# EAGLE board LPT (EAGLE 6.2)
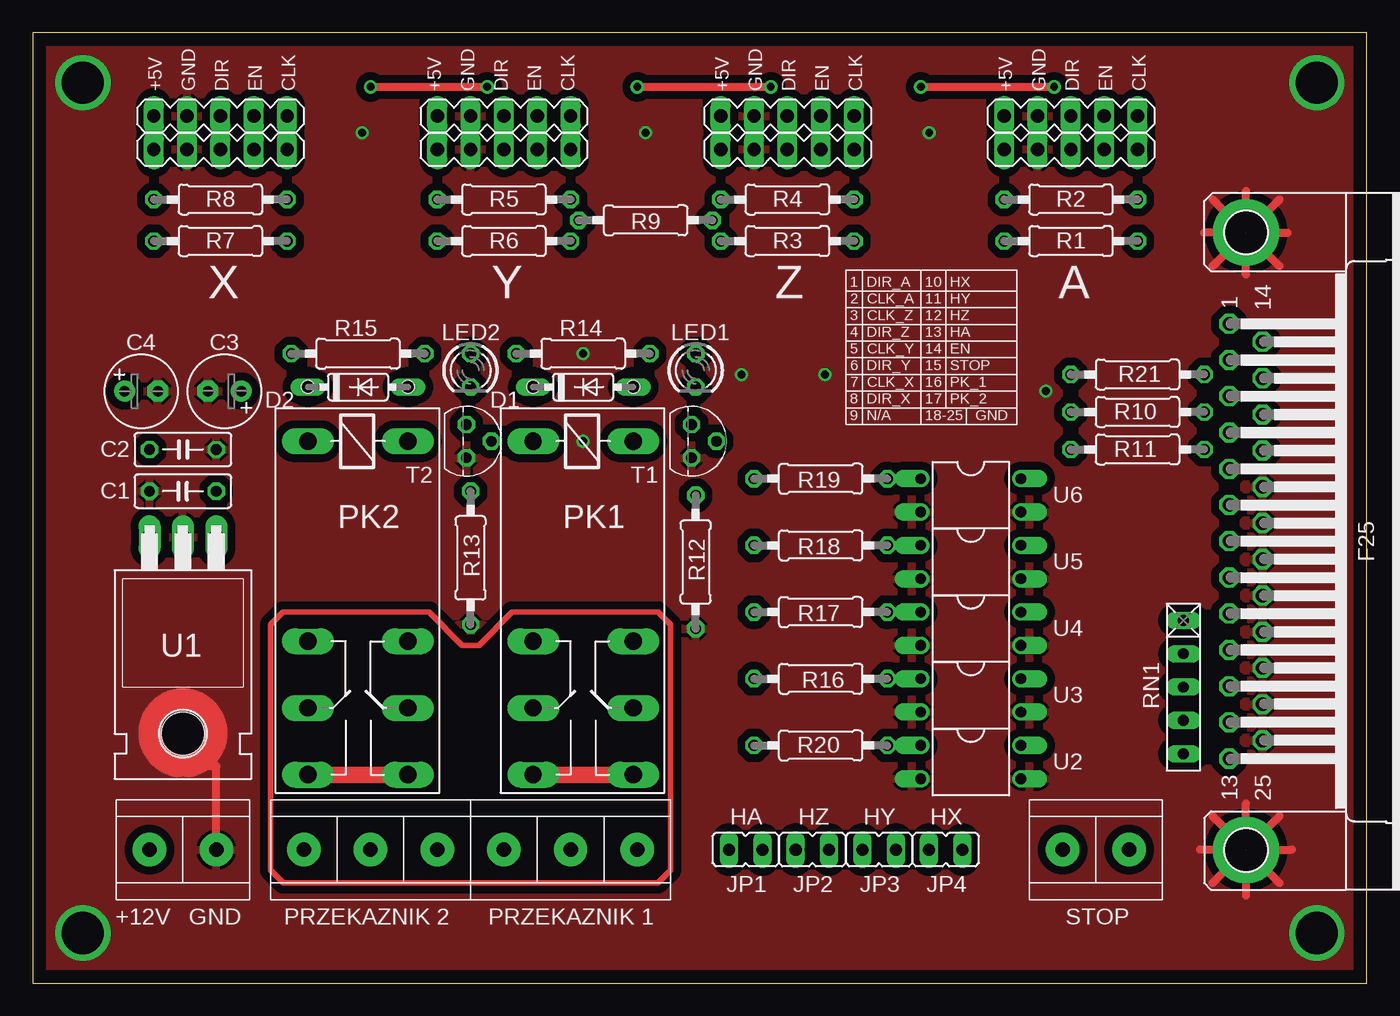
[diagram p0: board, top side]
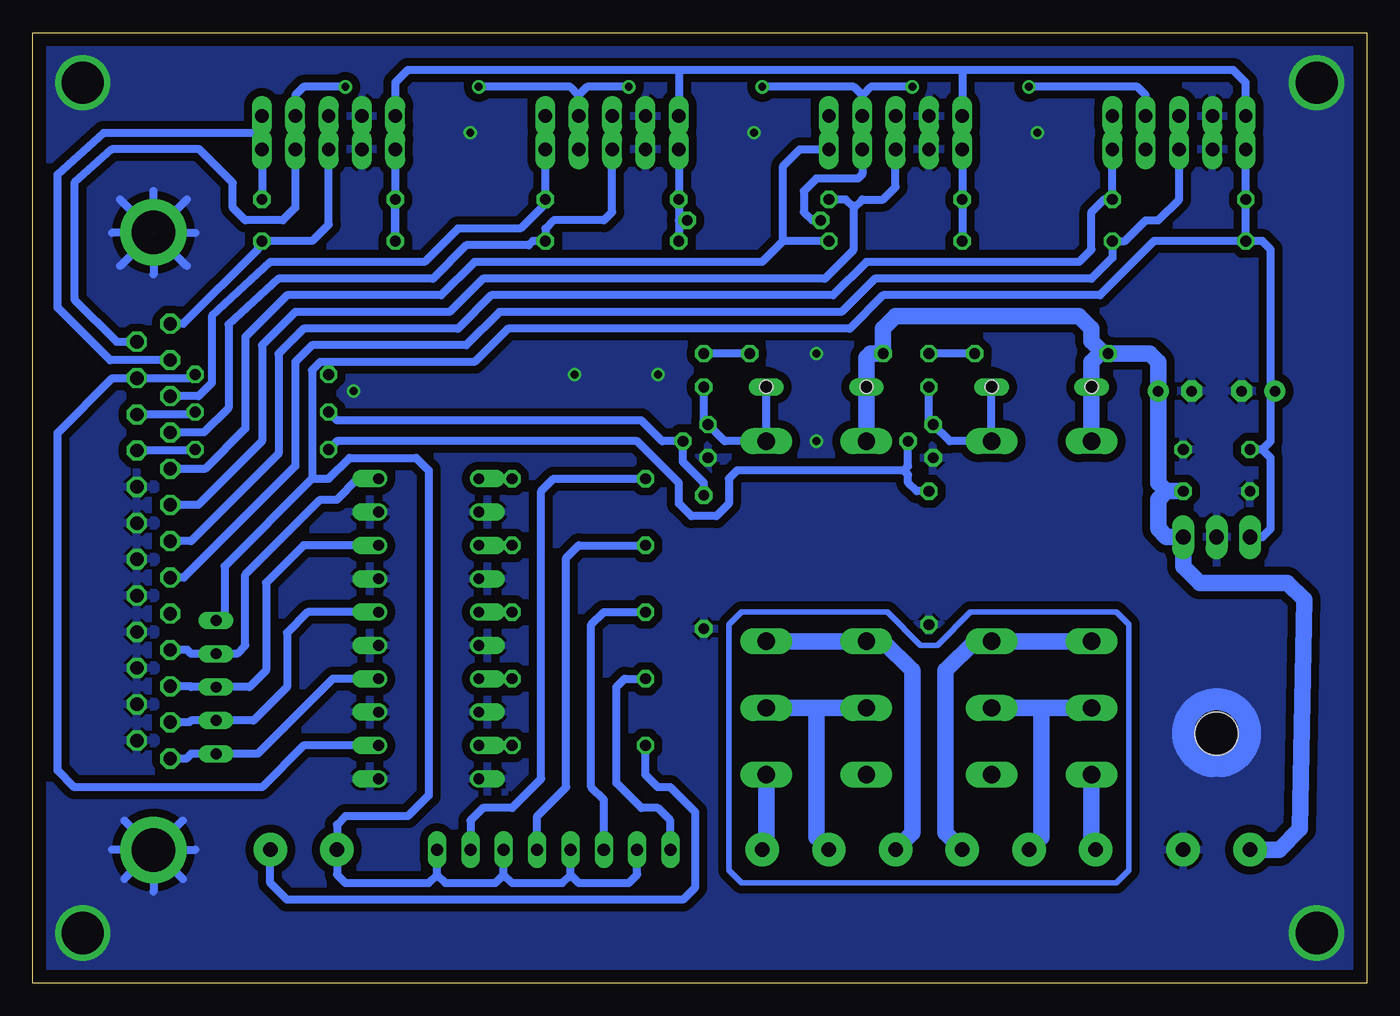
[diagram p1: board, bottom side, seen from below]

Size 101.59 x 72.38 mm. Coordinates in mm from the lower left corner, seen from the top.
Outline: 0,0 101.59,0 101.59,72.38 0,72.38 0,0
Copper layers (1*16): Top 0.035mm / dielectric 1.5mm / Bottom 0.035mm
Design rules: minimum track width 10mil, minimum drill 24mil, track to track 8mil, track to pad 8mil, pad to pad 8mil, via to via 8mil, smd to smd 8mil, copper to edge 40mil, drill to drill 8mil, minimum pad ring 10mil, minimum via ring 8mil, stop-mask expansion 4mil, vias tented up to drill 0mil, thermal gap 10mil
Holes 1 mm at 20.96,45.4 28.57,45.4 38.1,45.4 45.72,45.4

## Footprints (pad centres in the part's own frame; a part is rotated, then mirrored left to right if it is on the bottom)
MA05-1 = drill 1.016 long: 1 -5.08,0; 2 -2.54,0; 3 0,0; 4 2.54,0; 5 5.08,0
C050-025X075 = drill 0.813 octagon: 1 -2.54,0; 2 2.54,0
E2,5-6 = drill 0.813 pad 1.6: + -1.27,0 | drill 0.813 pad 1.6 octagon: - 1.27,0
DO35-7 = drill 0.813 long: A 3.81,0; C -3.81,0
JP1 = drill 0.914 long: 1 0,-1.27; 2 0,1.27
LED3MM = drill 0.813 octagon: A -1.27,0; K 1.27,0
F25HP = drill 1.016 octagon: 1 -16.561,-1.27; 2 -13.792,-1.27; 3 -11.049,-1.27; 4 -8.28,-1.27; 5 -5.512,-1.27; 6 -2.769,-1.27; 7 0,-1.27; 8 2.769,-1.27; 9 5.512,-1.27; 10 8.28,-1.27; 11 11.049,-1.27; 12 13.792,-1.27; 13 16.561,-1.27; 14 -15.189,1.27; 15 -12.421,1.27; 16 -9.652,1.27; 17 -6.909,1.27; 18 -4.14,1.27; 19 -1.372,1.27; 20 1.372,1.27; 21 4.14,1.27; 22 6.909,1.27; 23 9.652,1.27; 24 12.421,1.27; 25 15.189,1.27 | drill 3.302 pad 5.08: G1 -23.52,0; GND 23.52,0
F4052 = drill 1.321 long: 1 -3.81,3.81; 2 -3.81,-3.81; O1 11.43,-3.81; O2 11.43,3.81; P1 16.51,-3.81; P2 16.51,3.81; S1 21.59,-3.81; S2 21.59,3.81
0207/10 = drill 0.813 octagon: 1 -5.08,0; 2 5.08,0
RN-5 = drill 0.813 long: 1 -5.08,0; 2 -2.54,0; 3 0,0; 4 2.54,0; 5 5.08,0
TO92 = drill 0.813 octagon: 1 1.27,0; 2 0,1.905; 3 -1.27,0
TO220H = drill 1.118 long: 1 -2.54,-10.16; 2 0,-10.16; 3 2.54,-10.16 | hole 3.302: 0,4.826
DIL04 = drill 0.813 offset: 1 -1.27,-3.81; 2 1.27,-3.81; 3 1.27,3.81; 4 -1.27,3.81
AREK3 = drill 1.1 pad 2.54: P$1 0,0; P$2 -5.08,0; P$3 5.08,0
ARK2 = drill 1.1 pad 2.54: P$1 -2.54,0; P$2 2.54,0

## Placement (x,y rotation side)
A  [MA05-1]  79.06,63.5 0 top
C1  100nF  [C050-025X075]  11.43,37.46 180 top
C2  100nF  [C050-025X075]  11.43,40.64 0 top
C3  100uF  [E2,5-6]  14.61,45.09 180 top
C4  100uF  [E2,5-6]  8.25,45.09 0 top
D1  1N4148DO35-7  [DO35-7]  41.91,45.4 0 top
D2  1N4148DO35-7  [DO35-7]  24.77,45.4 0 top
JP1  [JP1]  54.29,10.16 270 top
JP2  [JP1]  59.37,10.16 270 top
JP3  [JP1]  64.45,10.16 270 top
JP4  [JP1]  69.53,10.16 270 top
LED1  [LED3MM]  50.48,46.67 270 top
LED2  [LED3MM]  33.34,46.67 270 top
LPT  [F25HP]  92.39,33.66 270 top
PK1  4052  [F4052]  41.91,37.46 270 top
PK2  4052  [F4052]  24.77,37.46 270 top
R1  [0207/10]  79.06,56.52 180 top
R2  [0207/10]  79.06,59.69 180 top
R3  [0207/10]  57.47,56.52 180 top
R4  [0207/10]  57.47,59.69 180 top
R5  [0207/10]  35.88,59.69 180 top
R6  [0207/10]  35.88,56.52 180 top
R7  [0207/10]  14.29,56.52 180 top
R8  [0207/10]  14.29,59.69 180 top
R9  [0207/10]  46.67,58.1 0 top
R10  4,7k  [0207/10]  84.14,43.5 180 top
R11  4,7k  [0207/10]  84.14,40.64 180 top
R12  10k  [0207/10]  50.48,32.07 90 top
R13  10k  [0207/10]  33.34,32.38 90 top
R14  1k  [0207/10]  41.91,47.94 180 top
R15  1k  [0207/10]  24.77,47.94 180 top
R16  330  [0207/10]  60.01,23.18 0 top
R17  330  [0207/10]  60.01,28.26 0 top
R18  330  [0207/10]  60.01,33.34 0 top
R19  330  [0207/10]  60.01,38.42 0 top
R20  330  [0207/10]  60.01,18.1 0 top
R21  4,7k  [0207/10]  84.14,46.35 180 top
RN1  4x4,7k  [RN-5]  87.63,22.54 270 top
S5  [MA05-1]  14.29,66.04 0 top
S6  [MA05-1]  35.88,66.04 0 top
S7  [MA05-1]  57.47,66.04 0 top
S8  [MA05-1]  79.06,66.04 0 top
T1  BC547  [TO92]  50.17,41.27 270 top
T2  BC547  [TO92]  33.02,41.27 270 top
U1  7805T  [TO220H]  11.43,23.81 180 top
U2  PC817  [DIL04]  71.44,16.83 270 top
U3  PC817  [DIL04]  71.44,21.91 270 top
U4  PC817  [DIL04]  71.44,26.99 270 top
U5  PC817  [DIL04]  71.44,32.07 270 top
U6  PC817  [DIL04]  71.44,37.15 270 top
U$2  AREK3  [AREK3]  40.96,10.16 180 top
U$3  AREK3  [AREK3]  25.72,10.16 0 top
U$5  ARK2  [ARK2]  80.96,10.16 180 top
U$7  ARK2  [ARK2]  11.43,10.16 0 top
X  [MA05-1]  14.29,63.5 0 top
Y  [MA05-1]  35.88,63.5 0 top
Z  [MA05-1]  57.47,63.5 0 top

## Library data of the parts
A S5-S8 X Y Z = con-lstb
C1-C4 R1-R21 = rcl
D1 D2 = diode
JP1-JP4 = jumper
LED1 LED2 = led
LPT = con-subd
PK1 PK2 = relay
RN1 = resistor-net
T1 T2 = transistor-npn
U1 = linear
U2-U6 = optocoupler
U$2 U$3 = arek3
U$5 U$7 = !ark2m

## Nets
GND: A.2 C1.2 C2.2 C3.- C4.- LPT.18 LPT.19 LPT.20 LPT.21 LPT.22 LPT.23 LPT.24 LPT.25 R12.1 R13.1 S5.2 S6.2 S7.2 S8.2 T1.1 T2.1 U1.2 U2.2 U2.3 U3.2 U3.3 U4.2 U4.3 U5.2 U5.3 U6.2 U6.3 U$7.P$2 X.2 Y.2 Z.2
N$1: D1.A LED1.K PK1.1 T1.3
N$2: D2.A LED2.K PK2.1 T2.3
N$3: LPT.5 R6.1 S6.5 Y.5
N$4: LPT.6 R5.1 S6.3 Y.3
N$5: LPT.8 R7.1 S5.3 X.3
N$6: LPT.4 R3.1 S7.3 Z.3
N$7: A.5 LPT.2 R2.1 S8.5
N$9: PK1.S1 PK1.S2 U$2.P$2
N$10: A.4 LPT.14 R9.1 S5.4 S6.4 S7.4 S8.4 X.4 Y.4 Z.4
N$11: A.3 LPT.1 R1.1 S8.3
N$12: LPT.7 R8.1 S5.5 X.5
N$13: LPT.3 R4.1 S7.5 Z.5
N$14: PK1.O1 PK1.O2 U$2.P$3
N$15: A.1 C2.1 C4.+ JP1.2 JP2.2 JP3.2 JP4.2 R1.2 R2.2 R3.2 R4.2 R5.2 R6.2 R7.2 R8.2 R9.2 R21.2 RN1.1 S5.1 S6.1 S7.1 S8.1 U1.3 U$5.P$2 X.1 Y.1 Z.1
N$16: R10.2 R12.2 T1.2
N$17: R11.2 R13.2 T2.2
N$18: LED1.A R14.1
N$19: LED2.A R15.1
N$20: LPT.16 R10.1
N$21: LPT.17 R11.1
N$24: LPT.15 R21.1 U2.4
N$25: LPT.10 RN1.2 U6.4
N$26: PK2.S1 PK2.S2 U$3.P$2
N$27: PK2.O1 PK2.O2 U$3.P$3
N$28: PK2.P1 PK2.P2 U$3.P$1
N$29: LPT.11 RN1.3 U5.4
N$30: LPT.12 RN1.4 U4.4
N$31: LPT.13 RN1.5 U3.4
N$32: R16.2 U3.1
N$33: R17.2 U4.1
N$34: R18.2 U5.1
N$35: R19.2 U6.1
N$36: JP3.1 R18.1
N$38: JP1.1 R16.1
N$39: JP2.1 R17.1
N$40: JP4.1 R19.1
N$42: C1.1 C3.+ D1.C D2.C PK1.2 PK2.2 R14.2 R15.2 U1.1 U$7.P$1
N$45: R20.2 U2.1
N$46: R20.1 U$5.P$1
N$47: PK1.P1 PK1.P2 U$2.P$1

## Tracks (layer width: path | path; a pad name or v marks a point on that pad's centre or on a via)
GND  (via drill 0.6, 3.2)  (3 unrouted)
  Top 0.61: 92.39,10.16 89.85,12.7 | 92.39,10.16 94.93,7.62 | 92.39,10.16 95.88,10.16 | 92.39,10.16 88.9,10.16 | 92.39,10.16 94.93,12.7 | 89.85,7.62 92.39,10.16 | 92.39,10.16 92.39,6.67 | 92.39,57.15 94.93,59.69 | 92.39,57.15 89.85,54.61 | 92.39,57.15 89.22,57.15 | 92.39,57.15 89.85,59.69 | 92.39,57.15 94.93,54.61 | 92.39,57.15 92.39,60.32 | 92.39,53.98 92.39,57.15 | 92.39,10.16 92.39,13.65 | 92.39,57.15 95.57,57.15 | U$7.P$2 13.97,16.51 11.75,16.51
  Top 1.676: 11.75,16.51 arc346 11.11,16.51
  Bottom 0.61: Z.2 S7.2 | A.2 S8.2 | Y.2 S6.2 | 92.39,10.16 95.57,10.16 | 92.39,10.16 89.22,10.16 | 92.39,10.16 92.39,6.99 | 92.39,10.16 94.61,7.94 | 92.39,10.16 90.17,12.38 | 92.39,10.16 92.39,12.38 | 92.39,10.16 94.61,12.38 | 90.17,7.94 92.39,10.16 | 92.39,57.15 92.39,53.98 | 92.39,57.15 92.39,60.32 | 92.39,57.15 95.57,57.15 | 92.39,57.15 89.22,57.15 | 92.39,57.15 94.93,54.61 | 92.39,57.15 89.85,59.69 | 89.85,54.61 92.39,57.15 | 92.39,57.15 94.93,59.69
  Bottom 1.676: 11.11,16.51 arc-346 11.75,16.51
  other vias: 97.79,3.81 97.79,68.58 3.81,68.58 68.26,64.77 46.67,64.77 25.08,64.77 3.81,3.81 77.15,45.09 41.91,41.27 41.91,47.94 53.97,46.35 60.33,46.35
  pour Bottom (isolate 0.61, rank 5): 101.92,-0.32 101.92,72.71 -0.32,72.71 -0.32,-0.32
  pour Top (isolate 0.61): 101.92,-0.32 101.92,72.71 -0.32,72.71 -0.32,-0.32
N$1
  Bottom 0.61: D1.A PK1.1 48.89,41.27 T1.3 50.48,42.86 LED1.K
N$2
  Bottom 0.61: D2.A PK2.1 31.75,41.27 T2.3 33.34,42.86 LED2.K
N$3
  Bottom 0.61: R6.1 44.45,56.52 | S6.5 Y.5 43.18,63.5 44.45,62.23 44.45,56.52 | 44.45,56.52 46.04,54.93 67.94,54.93 70.49,52.39 82.23,52.39 85.41,49.21 85.41,42.23 88.47,39.17 LPT.5
N$4
  Bottom 0.61: 39.05,59.05 39.05,55.88 41.28,53.66 67.31,53.66 69.85,51.12 81.6,51.12 84.14,48.58 84.14,41.27 88.99,36.42 LPT.6 | 39.05,59.05 38.42,59.69 36.83,59.69 35.88,60.64 Y.3 | 39.05,59.05 39.69,59.69 R5.1 | Y.3 S6.3 Y.3
N$5
  Bottom 0.61: LPT.8 90.08,30.89 81.6,39.37 81.6,47.31 80.33,48.58 68.58,48.58 66.04,51.12 40,51.12 37.46,53.66 20.96,53.66 19.37,55.24 R7.1 18.41,56.52 16.83,58.1 15.87,58.1 14.29,59.69 X.3 S5.3
N$6
  Bottom 0.61: S7.3 Z.3 57.47,58.74 58.1,58.1 61.91,58.1 62.55,57.47 R3.1 63.5,56.52 63.82,56.2 68.58,56.2 71.12,53.66 82.87,53.66 86.68,50.16 86.68,43.81 88.56,41.93 LPT.4
N$7
  Bottom 0.61: R2.1 A.5 84.14,64.77 | 84.14,64.77 S8.5 | LPT.2 95.71,47.45 99.69,51.43 99.69,61.59 96.2,64.77 84.14,64.77
N$9
  Top 1.27: PK1.S1 PK1.S2
  Bottom 1.27: PK1.S2 45.72,10.48 U$2.P$2
N$10  (via drill 0.6)
  Top 0.61: v67.63,68.26 v77.79,68.26 | v46.04,68.26 v56.2,68.26 | v25.72,68.26 v34.61,68.26
  Bottom 0.61: X.4 S5.4 16.83,67.63 17.46,68.26 v25.72,68.26 | S8.4 A.4 | Z.4 S7.4 60.01,67.63 | v34.61,68.26 37.78,68.26 38.42,67.63 | 38.42,67.63 S6.4 Y.4 38.42,61.59 38.74,61.28 41.91,61.28 42.86,60.32 42.86,58.74 42.23,58.1 R9.1 | 38.42,67.63 39.05,68.26 v46.04,68.26 | v56.2,68.26 59.37,68.26 60.01,67.63 | S8.4 A.4 | S8.4 81.6,67.63 80.96,68.26 v77.79,68.26 | v67.63,68.26 60.64,68.26 60.01,67.63 | LPT.14 95.2,48.84 98.43,52.07 98.43,60.96 95.57,63.5 88.9,63.5 86.36,60.96 86.36,59.05 85.41,58.1 82.55,58.1 81.6,59.05 A.4
N$11
  Bottom 0.61: A.3 S8.3 A.3 | A.3 79.06,57.79 80.33,56.52 R1.1 84.46,56.2 84.46,55.88 90.12,50.22 LPT.1
N$12
  Bottom 0.61: S5.5 X.5 R8.1 20,59.69 20.96,58.74 20.96,55.88 21.91,54.93 38.1,54.93 40.64,52.39 66.68,52.39 69.22,49.85 80.96,49.85 82.87,47.94 82.87,40.32 89.53,33.66 LPT.7
N$13
  Bottom 0.61: Z.5 S7.5 | R4.1 Z.5 | R4.1 Z.5 | LPT.3 88.96,44.7 87.95,45.72 87.95,50.8 83.5,54.93 71.75,54.93 69.22,57.47 64.45,57.47 62.55,59.37 R4.1
N$14
  Bottom 1.27: PK1.O2 PK1.O1 36.83,26.03 34.61,23.81 34.61,11.43 U$2.P$3
N$15
  Bottom 0.61: R6.2 R5.2 Y.1 | R2.2 R1.2 A.1 S8.1 73.98,68.58 73.02,69.53 52.39,69.53 | X.1 S5.1 | S6.1 Y.1 | X.1 S5.1 | S6.1 Y.1 | 52.39,58.1 R4.2 Z.1 S7.1 52.39,69.53 | S5.1 9.21,68.58 10.16,69.53 30.8,69.53 | 30.8,69.53 52.39,69.53 | 30.8,69.53 S6.1 | X.1 R8.2 R7.2 | 52.39,58.1 R9.2 | 52.39,58.1 R3.2 | RN1.1 86.99,27.62 86.99,31.75 80.33,38.42 | R7.2 16.19,56.52 20.32,52.39 36.83,52.39 39.37,49.85 65.4,49.85 67.94,47.31 79.06,47.31 | U1.3 7.94,33.97 7.3,34.61 7.3,40 7.94,40.64 | 7.94,40.64 C2.1 | 7.94,40.64 7.3,41.27 7.3,44.77 C4.+ 6.99,45.4 7.3,45.72 7.3,55.88 7.94,56.52 R7.2 | 79.06,47.31 R21.2 | 80.33,38.42 80.33,46.67 79.69,47.31 79.06,47.31 | 60.64,8.26 JP2.2 | JP1.2 55.56,8.26 56.2,7.62 60.01,7.62 60.64,8.26 | 60.64,8.26 61.28,7.62 65.09,7.62 65.72,8.26 | 65.72,8.26 JP3.2 | 65.72,8.26 66.36,7.62 70.17,7.62 70.8,8.26 | 70.8,8.26 JP4.2 | 70.8,8.26 71.44,7.62 77.79,7.62 78.42,8.26 U$5.P$2 78.42,12.06 77.79,12.7 73.02,12.7 71.44,14.29 71.44,39.05 72.39,40 77.47,40 79.06,38.42 80.33,38.42
N$16
  Bottom 0.61: R10.2 78.42,42.86 55.25,42.86 53.66,41.27 T1.2 52.07,39.69 50.48,38.1 R12.2
N$17
  Bottom 0.61: R11.2 78.42,41.27 55.56,41.27 52.39,38.1 52.39,36.51 51.43,35.56 49.53,35.56 48.58,36.51 48.58,38.42 47.94,39.05 35.24,39.05 | R13.2 34.29,37.46 34.93,38.1 34.93,38.73 35.24,39.05 | T2.2 34.93,39.37 35.24,39.05
N$18
  Bottom 0.61: R14.1 LED1.A
N$19
  Bottom 0.61: R15.1 LED2.A
N$20
  Bottom 0.61: LPT.16 89.34,43.31 R10.1
N$21
  Bottom 0.61: LPT.17 89.29,40.56 R11.1
N$22
  Bottom 0.406: 33.97,25.72 36.51,28.26 47.63,28.26 48.58,27.3 48.58,8.57 47.63,7.62 19.05,7.62 18.1,8.57 18.1,27.3 19.05,28.26 30.16,28.26 32.7,25.72 33.97,25.72
N$24
  Bottom 0.61: U2.4 80.96,18.1 84.14,14.92 98.43,14.92 99.69,16.19 99.69,41.91 95.53,46.08 LPT.15 89.5,46.08 R21.1
N$25
  Bottom 0.61: LPT.10 89.83,25.38 89.53,25.08 RN1.2 86.04,25.08 85.41,25.72 85.41,31.12 79.69,36.83 78.42,36.83 76.83,38.42 U6.4
N$26
  Top 1.27: PK2.S1 PK2.S2
  Bottom 1.27: PK2.S1 20.96,10.48 U$3.P$2
N$27
  Bottom 1.27: PK2.O1 PK2.O2 29.84,26.03 32.07,23.81 32.07,11.43 U$3.P$3
N$28
  Bottom 1.27: 24.77,20.95 PK2.P1 | 24.77,20.95 PK2.P2 | 24.77,20.95 24.77,11.11 U$3.P$1
N$29
  Bottom 0.61: LPT.11 89.6,22.61 89.53,22.54 RN1.3 85.09,22.54 83.82,23.81 83.82,30.48 80.96,33.34 U5.4
N$30
  Bottom 0.61: LPT.12 89.67,19.86 89.53,20 RN1.4 84.77,20 82.23,22.54 82.23,26.67 80.64,28.26 U4.4
N$31
  Bottom 0.61: LPT.13 89.9,17.09 89.53,17.46 RN1.5 84.46,17.46 78.74,23.18 U3.4
N$32
  Bottom 0.61: R16.2 U3.1
N$33
  Bottom 0.61: R17.2 U4.1
N$34
  Bottom 0.61: R18.2 U5.1
N$35
  Bottom 0.61: R19.2 U6.1
N$36
  Bottom 0.61: R18.1 60.01,33.34 60.96,32.38 60.96,14.92 63.18,12.7 JP3.1
N$38
  Bottom 0.61: R16.1 56.51,23.18 57.15,22.54 57.15,15.24 55.25,13.33 53.97,13.33 53.02,12.38 JP1.1
N$39
  Bottom 0.61: R17.1 58.1,28.26 59.06,27.3 59.06,14.92 58.1,13.97 JP2.1
N$40
  Bottom 0.61: R19.1 61.91,38.42 62.86,37.46 62.86,15.56 65.09,13.33 67.31,13.33 68.26,12.38 JP4.1
N$42
  Bottom 0.61: D2.C PK2.2 | D1.C PK1.2
  Bottom 1.27: U$7.P$1 6.67,10.16 5.08,11.75 4.76,29.21 6.03,30.48 12.7,30.48 13.97,31.75 U1.1 15.24,33.97 15.87,34.61 15.87,36.83 15.24,37.46 | 15.24,37.46 C1.1 | 15.24,37.46 15.87,38.1 C3.+ 15.87,47.31 16.51,47.94 R15.2 | R15.2 20.32,47.94 20.96,47.31 D2.C PK2.2 | PK1.2 D1.C 38.1,47.62 37.78,47.94 R14.2 36.83,49.85 35.88,50.8 21.91,50.8 20.96,49.85 20.96,48.89 20,47.94 R15.2
N$44
  Top 0.406: 18.1,8.57 19.05,7.62 47.63,7.62 48.58,8.57 48.58,27.3 47.63,28.26 36.51,28.26 33.97,25.72 32.7,25.72 30.16,28.26 19.05,28.26 18.1,27.3 18.1,8.57
N$45
  Bottom 0.61: R20.2 U2.1
N$46
  Bottom 0.61: R20.1 54.93,15.88 53.97,14.92 53.02,14.92 51.12,13.02 51.12,7.3 52.07,6.35 82.23,6.35 83.5,7.62 U$5.P$1
N$47
  Bottom 1.27: 41.91,20.95 PK1.P2 | 41.91,20.95 PK1.P1 | 41.91,20.95 41.91,11.11 U$2.P$1

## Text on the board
tPlace: +5V | GND | DIR | EN | CLK | +5V | GND | DIR | EN | CLK | +5V | GND | DIR | EN | CLK | +5V | GND | DIR | EN | CLK | 1 | DIR_A | 10 | HX | 2 | CLK_A | 11 | HY | 3 | CLK_Z | 12 | HZ | 4 | DIR_Z | 13 | HA | 5 | CLK_Y | 14 | EN | 6 | DIR_Y | 15 | STOP | 7 | CLK_X | 16 | PK_1 | 8 | DIR_X | 17 | PK_2 | 9 | N/A | 18-25 | GND | HA | HZ | HY | HX | +12V | GND | PRZEKAZNIK 2 | PRZEKAZNIK 1 | STOP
